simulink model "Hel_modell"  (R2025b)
settings: Solver=VariableStepAuto  StartTime=0.0  StopTime=10.0  RelTol=1e-3
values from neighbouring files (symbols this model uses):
  AFs = 14.6    [Lektion_2.m]
  eta_vol = 0.8    [Lektion_2.m]
  Je = 0.1    [Lektion_2.m]
  Ki = 0.1    [Lektion_2.m]
  Kp = 0    [Lektion_2.m]
  lamda_eg_init = 1    [Lektion_2.m]
  lamda_s_init = 1    [Lektion_2.m]
  m_dot_a_end = 18*1e-3    (= 0.018)    [Lektion_2.m]
  m_dot_a_start = 12*1e-3    (= 0.012)    [Lektion_2.m]
  m_dot_fi_start = m_dot_a_start/AFs    (= 0.000821917808219)    [Lektion_2.m]
  n_cyl = 4    [Lektion_2.m]
  N_init = 3000/60    (= 50)    [Lektion_2.m]
  n_r = 2    [Lektion_2.m]
  p_im_init = 40*1e3    (= 40000)    [Lektion_2.m]
  R = 280    [Lektion_2.m]
  T_i = 320    [Lektion_2.m]
  tau_d = 0.2    [Lektion_2.m]
  tau_mix = 0.14    [Lektion_2.m]
  tau_sensor = 0.05    [Lektion_2.m]
  tau_th = 1/0.1    (= 10)    [Lektion_2.m]
  V_d = 0.55/1e3    (= 0.00055)    [Lektion_2.m]
  V_i = 2/1e3    (= 0.002)    [Lektion_2.m]

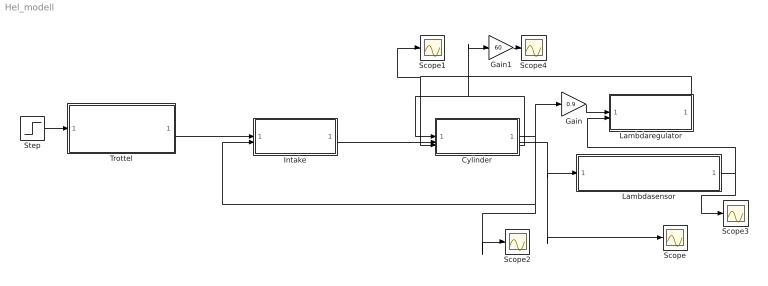
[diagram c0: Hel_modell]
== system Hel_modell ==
  Cylinder : Subsystem
  Gain : Gain  Gain=0.9
  Gain1 : Gain  Gain=60
  Intake : Subsystem
  Lambdaregulator : Subsystem
  Lambdasensor : Subsystem
  Scope{,1..4} (5 alike) : Scope
  Step : Step  Time=5  Before=m_dot_a_start  After=m_dot_a_end  SampleTime=0
  Trottel : Subsystem
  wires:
  Cylinder/1(m_ac [kg/s]) -> Scope2/1, Intake/2(m_ac [kg/s]), Gain/1
  Step/1 -> Trottel/1(m_at,raf [kg/s])
  Trottel/1(m_at [kg/s]) -> Intake/1(m_at [kg/s])
  Intake/1(p_im [Pa]) -> Cylinder/2(p_im [Pa])
  Cylinder/3(N_e [rps]) -> Gain1/1, Cylinder/1(N [rps])
  Lambdaregulator/1(m_fi [kg/s]) -> Cylinder/3(m_fi [kg/s]), Scope1/1
  Cylinder/2(lambda_c [-]) -> Scope/1, Lambdasensor/1(lambda_c [-])
  Lambdasensor/1(lambda_d [-]) -> Scope3/1, Lambdaregulator/2(lambda_d [-])
  Gain/1 -> Lambdaregulator/1(m_ac_mod)
  Gain1/1 -> Scope4/1

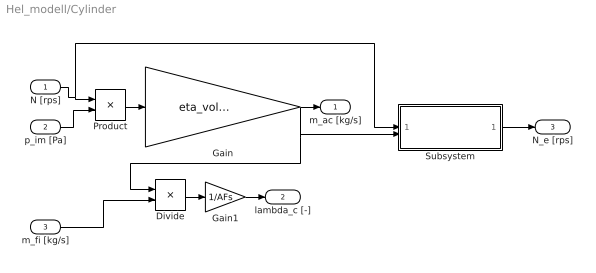
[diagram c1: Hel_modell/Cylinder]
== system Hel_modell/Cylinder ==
  N [rps] : Inport
  p_im [Pa] : Inport  Port=2
  m_fi [kg/s] : Inport  Port=3
  Divide : Product  Inputs=*/
  Gain : Gain  Gain=eta_vol*V_d*n_cyl/(n_r*R*T_i)
  Gain1 : Gain  Gain=1/AFs
  Product : Product
  Subsystem : Subsystem
  m_ac [kg/s] : Outport
  lambda_c [-] : Outport  Port=2
  N_e [rps] : Outport  Port=3
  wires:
  N [rps]/1 -> Subsystem/1(N [rps]), Product/1
  p_im [Pa]/1 -> Product/2
  Product/1 -> Gain/1
  Gain/1 -> Divide/1, Subsystem/2(m_ac [kg/s]), m_ac [kg/s]/1
  m_fi [kg/s]/1 -> Divide/2
  Divide/1 -> Gain1/1
  Gain1/1 -> lambda_c [-]/1
  Subsystem/1(N_e [rps]) -> N_e [rps]/1

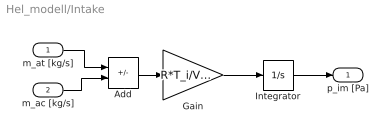
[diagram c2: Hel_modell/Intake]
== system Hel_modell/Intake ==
  m_at [kg/s] : Inport
  m_ac [kg/s] : Inport  Port=2
  Add : Sum  Inputs=+-
  Gain : Gain  Gain=R*T_i/V_i
  Integrator : Integrator  InitialCondition=p_im_init
  p_im [Pa] : Outport
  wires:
  Integrator/1 -> p_im [Pa]/1
  Gain/1 -> Integrator/1
  m_ac [kg/s]/1 -> Add/2
  m_at [kg/s]/1 -> Add/1
  Add/1 -> Gain/1

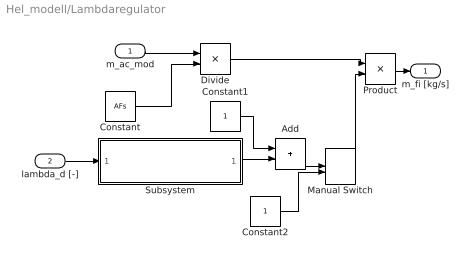
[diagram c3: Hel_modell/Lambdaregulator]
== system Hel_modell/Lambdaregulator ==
  m_ac_mod : Inport
  lambda_d [-] : Inport  Port=2
  Add : Sum
  Constant : Constant  Value=AFs
  Constant1 : Constant
  Constant2 : Constant
  Divide : Product  Inputs=*/
  Manual Switch : ManualSwitch
  Product : Product
  Subsystem : Subsystem
  m_fi [kg/s] : Outport
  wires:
  m_ac_mod/1 -> Divide/1
  Constant/1 -> Divide/2
  Constant1/1 -> Add/1
  Divide/1 -> Product/1
  Product/1 -> m_fi [kg/s]/1
  Subsystem/1("Lambda_controlled ") -> Add/2
  lambda_d [-]/1 -> Subsystem/1(lambda_d)
  Add/1 -> Manual Switch/1
  Manual Switch/1 -> Product/2
  Constant2/1 -> Manual Switch/2

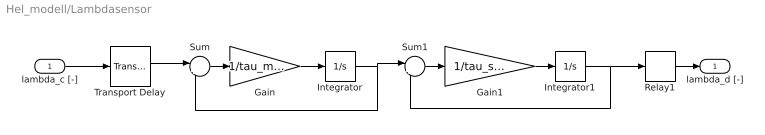
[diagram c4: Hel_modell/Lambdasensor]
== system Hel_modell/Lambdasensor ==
  lambda_c [-] : Inport
  Gain : Gain  Gain=1/tau_mix
  Gain1 : Gain  Gain=1/tau_sensor
  Integrator : Integrator  InitialCondition=lamda_eg_init
  Integrator1 : Integrator  InitialCondition=lamda_s_init
  Relay1 : Relay  OnSwitchValue=1+eps  OffSwitchValue=1-eps  OffOutputValue=-1
  Sum : Sum  Inputs=|+-
  Sum1 : Sum  Inputs=|+-
  Transport Delay : TransportDelay  DelayTime=tau_d  InitialOutput=0.8
  lambda_d [-] : Outport
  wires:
  lambda_c [-]/1 -> Transport Delay/1
  Transport Delay/1 -> Sum/1
  Gain/1 -> Integrator/1
  Sum/1 -> Gain/1
  Integrator/1 -> Sum/2, Sum1/1
  Sum1/1 -> Gain1/1
  Gain1/1 -> Integrator1/1
  Integrator1/1 -> Relay1/1, Sum1/2
  Relay1/1 -> lambda_d [-]/1

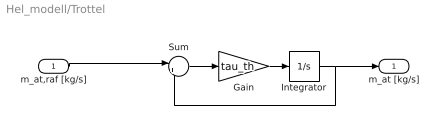
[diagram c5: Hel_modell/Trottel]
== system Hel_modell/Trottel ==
  m_at,raf [kg/s] : Inport
  Gain : Gain  Gain=tau_th
  Integrator : Integrator  InitialCondition=m_dot_a_start
  Sum : Sum  Inputs=|+-
  m_at [kg/s] : Outport
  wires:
  Sum/1 -> Gain/1
  Integrator/1 -> m_at [kg/s]/1, Sum/2
  m_at,raf [kg/s]/1 -> Sum/1
  Gain/1 -> Integrator/1

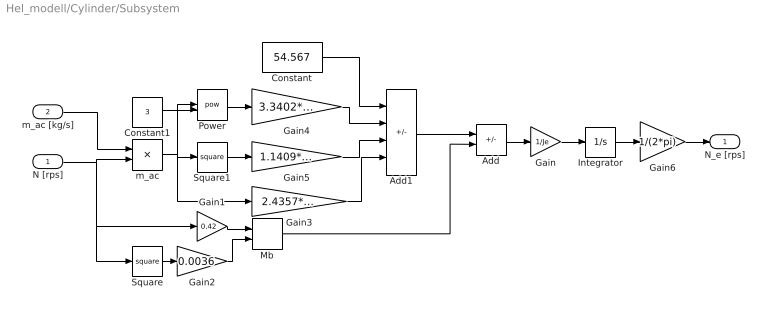
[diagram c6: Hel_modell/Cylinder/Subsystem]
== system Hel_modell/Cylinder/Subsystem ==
  N [rps] : Inport
  m_ac [kg/s] : Inport  Port=2
  Add : Sum  Inputs=+-
  Add1 : Sum  Inputs=-+-+
  Constant : Constant  Value=54.567
  Constant1 : Constant  Value=3
  Gain : Gain  Gain=1/Je
  Gain1 : Gain  Gain=0.42
  Gain2 : Gain  Gain=0.0036
  Gain3 : Gain  Gain=2.4357*10^5
  Gain4 : Gain  Gain=3.3402*10^10
  Gain5 : Gain  Gain=1.1409*10^2
  Gain6 : Gain  Gain=1/(2*pi)
  Integrator : Integrator  InitialCondition=N_init*2*pi
  Mb : Sum
  Power : Math  Operator=pow
  Square : Math  Operator=square
  Square1 : Math  Operator=square
  m_ac : Product  Inputs=*/
  N_e [rps] : Outport
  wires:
  m_ac [kg/s]/1 -> m_ac/1
  N [rps]/1 -> Gain1/1, Square/1, m_ac/2
  Gain/1 -> Integrator/1
  Gain1/1 -> Mb/1
  Gain2/1 -> Mb/2
  Square/1 -> Gain2/1
  Add/1 -> Gain/1
  Mb/1 -> Add/2
  m_ac/1 -> Power/1, Gain3/1, Square1/1
  Square1/1 -> Gain5/1
  Add1/1 -> Add/1
  Constant1/1 -> Power/2
  Power/1 -> Gain4/1
  Constant/1 -> Add1/1
  Gain4/1 -> Add1/2
  Gain5/1 -> Add1/3
  Gain3/1 -> Add1/4
  Integrator/1 -> Gain6/1
  Gain6/1 -> N_e [rps]/1

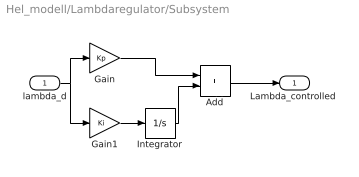
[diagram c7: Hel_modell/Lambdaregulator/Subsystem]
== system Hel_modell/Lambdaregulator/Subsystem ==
  lambda_d : Inport
  Add : Sum
  Gain : Gain  Gain=Kp
  Gain1 : Gain  Gain=Ki
  Integrator : Integrator  InitialCondition=m_dot_fi_start
  "Lambda_controlled " : Outport
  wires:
  Add/1 -> "Lambda_controlled "/1
  Gain1/1 -> Integrator/1
  Integrator/1 -> Add/2
  lambda_d/1 -> Gain/1, Gain1/1
  Gain/1 -> Add/1
